TYPE E_AnalysisIDs :
(
	(* analysis chain *)
	eID_Source := 1,
	eID_RainflowCounting,
	eID_MinersRule_RFC,
	eID_MeanStressCorrection,
	eID_MinersRule_MSC,
	eID_Sink_RFC,
	eID_Sink_MSC,
	eID_Sink_MR_RFC,
	eID_Sink_MR_MSC
	
) UDINT;
END_TYPE
